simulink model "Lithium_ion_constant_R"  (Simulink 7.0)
settings: Solver=ode23tb  StartTime=0.0  StopTime=10000  RelTol=1e-4
InitFcn:
  | load('CGR18650CG_data.mat');
undefined symbols (not defined in the file or in its folder): plecs
libraries: plecslib x2

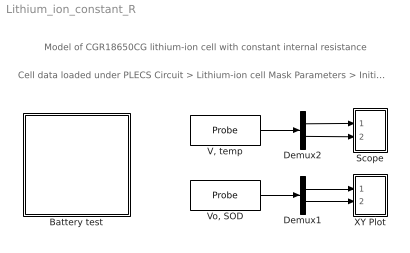
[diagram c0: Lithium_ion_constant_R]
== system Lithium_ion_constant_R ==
  note: Model of CGR18650CG lithium-ion cell with constant internal resistance
  note: Cell data loaded under PLECS Circuit > Lithium-ion cell Mask Parameters > Initialization
  Battery test : Subsystem  LoadFcn=plecs('sl', 200);  InitFcn=plecs('sl', 214);  StartFcn=plecs('sl', 208);  StopFcn=plecs('sl', 209);  mask(PlecsCircuit){PLECSData=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}
      mask prompts: PLECSData "PLECS Data (Do not delete or modify!)"
      mask init:
      | % PLACE CUSTOM INITIALIZATIONS ABOVE
      | % DO NOT REMOVE
      | plecs('sl', 215);
      | % DO NOT REMOVE
  Demux1 : Demux  Outputs=2
  Demux2 : Demux  Outputs=2
  Scope : Subsystem  LoadFcn=plecs('sl', 300);  StartFcn=plecs('sl', 308);  StopFcn=plecs('sl', 309);  mask{Settings=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}
      mask init:
      | plecsedit('sl', 315);
  "V, temp" : plecslib/Probe  SystemSampleTime=-1  tagno=1
  "Vo, SOD" : plecslib/Probe  SystemSampleTime=-1  tagno=3
  XY Plot : Subsystem  LoadFcn=plecs('sl', 317);  StartFcn=plecs('sl', 308);  StopFcn=plecs('sl', 309);  mask{Settings=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}
      mask init:
      | plecs('sl', 315);
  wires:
  "Vo, SOD"/1 -> Demux1/1
  Demux1/1 -> XY Plot/1(1)
  Demux1/2 -> XY Plot/2(2)
  "V, temp"/1 -> Demux2/1
  Demux2/1 -> Scope/1(1)
  Demux2/2 -> Scope/2(2)

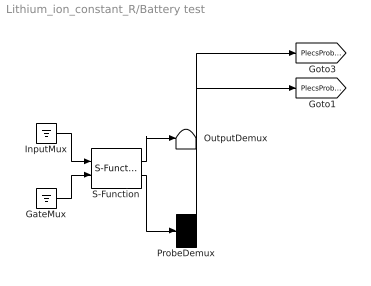
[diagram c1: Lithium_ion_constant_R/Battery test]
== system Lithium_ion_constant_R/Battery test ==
  " GateMux " : Ground
  " InputMux " : Ground
  " OutputDemux " : Terminator
  " ProbeDemux " : Demux  Outputs=[ 2 2 ]
  " S-Function " : S-Function  FunctionName=plecs
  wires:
  " S-Function "/1 -> " OutputDemux "/1
  " InputMux "/1 -> " S-Function "/1
  " GateMux "/1 -> " S-Function "/2
  " S-Function "/2 -> " ProbeDemux "/1
  " ProbeDemux "/1 -> [PlecsProbe3]
  " ProbeDemux "/2 -> [PlecsProbe1]

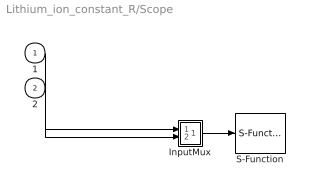
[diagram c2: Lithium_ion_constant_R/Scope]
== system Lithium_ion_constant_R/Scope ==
  1 : Inport  OutDataType=sfix(16)  OutScaling=2^0
  2 : Inport  Port=2  OutDataType=sfix(16)  OutScaling=2^0
  " InputMux " : Subsystem
  " S-Function " : S-Function  FunctionName=plecs
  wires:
  " InputMux "/1(Out) -> " S-Function "/1
  1/1 -> " InputMux "/1(In1)
  2/1 -> " InputMux "/2(In2)

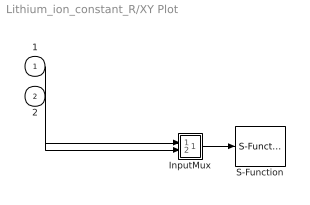
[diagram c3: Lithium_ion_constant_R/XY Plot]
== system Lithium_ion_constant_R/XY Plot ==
  1 : Inport
  2 : Inport  Port=2
  " InputMux " : Subsystem
  " S-Function " : S-Function  FunctionName=plecs
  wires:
  2/1 -> " InputMux "/1(In1)
  1/1 -> " InputMux "/2(In2)
  " InputMux "/1(Out) -> " S-Function "/1

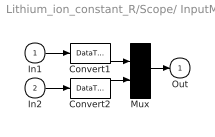
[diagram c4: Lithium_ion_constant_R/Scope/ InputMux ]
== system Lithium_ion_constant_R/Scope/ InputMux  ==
  In1 : Inport  OutDataType=sfix(16)  OutScaling=2^0
  In2 : Inport  Port=2  OutDataType=sfix(16)  OutScaling=2^0
  Convert1 : DataTypeConversion  OutDataType=sfix(16)  OutScaling=2^0
  Convert2 : DataTypeConversion  OutDataType=sfix(16)  OutScaling=2^0
  Mux : Mux  Inputs=2
  Out : Outport  OutDataType=sfix(16)  OutScaling=2^0
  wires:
  Mux/1 -> Out/1
  In1/1 -> Convert1/1
  In2/1 -> Convert2/1
  Convert1/1 -> Mux/1
  Convert2/1 -> Mux/2

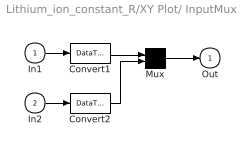
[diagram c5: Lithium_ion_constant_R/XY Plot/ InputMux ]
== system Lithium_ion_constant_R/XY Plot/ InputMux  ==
  In1 : Inport
  In2 : Inport  Port=2
  Convert1 : DataTypeConversion
  Convert2 : DataTypeConversion
  Mux : Mux  Inputs=2
  Out : Outport
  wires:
  Convert2/1 -> Mux/2
  In2/1 -> Convert2/1
  Convert1/1 -> Mux/1
  In1/1 -> Convert1/1
  Mux/1 -> Out/1
